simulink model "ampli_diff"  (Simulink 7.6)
settings: Solver=ode15s  StartTime=0.0  StopTime=.2  RelTol=1e-3
StopFcn:
  | close all, clc
  | load  ES_ampli_diff.mat
  | plot(x(1,:),x(2,:))
  | hold on
  | plot(x(1,:),x(3,:))
  | plot(x(1,:),x(4,:))
  | grid
  | title('Tensions d''entrée et de sortie - Ampli différentiel')
  | xlabel('temps')
libraries: fl_lib x13, nesl_utility x4

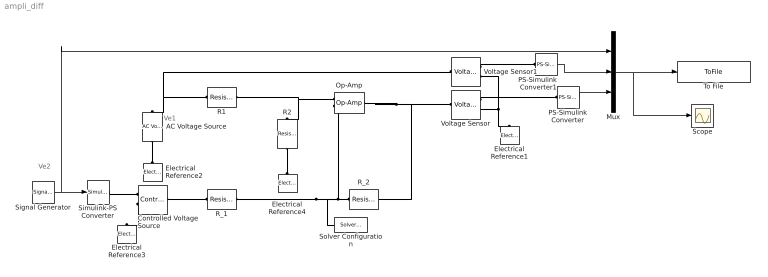
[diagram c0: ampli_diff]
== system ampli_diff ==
  note: Ve1
  note: Ve2
  AC Voltage Source : fl_lib/Electrical/Electrical Sources/AC Voltage Source  DialogController=NetworkEngine.DynNeDlgSource  SystemSampleTime=-1  amp=10 V  shift=2*pi/3 rad  omega=10 Hz  i_Log=off  v_Log=off  LocalVarNames=|current|voltage|power  LocalVarDescs=|Current (A)|Voltage (V)|Power (W)  LocalVarLogging=[0 0 0]
  Controlled Voltage Source : fl_lib/Electrical/Electrical Sources/Controlled Voltage Source  DialogController=NetworkEngine.DynNeDlgSource  SystemSampleTime=-1  i_Log=off  v_Log=off  LocalVarNames=|i|v  LocalVarDescs=|i|v  LocalVarLogging=[0 0]
  Electrical Reference{1..4} (4 alike) : fl_lib/Electrical/Electrical Elements/Electrical Reference  DialogController=NetworkEngine.DynNeDlgSource  SystemSampleTime=-1  i_Log=off  LocalVarNames=|i  LocalVarDescs=|i  LocalVarLogging=[]
  Mux : Mux  Inputs=3
  Op-Amp : fl_lib/Electrical/Electrical Elements/Op-Amp  DialogController=NetworkEngine.DynNeDlgSource  SystemSampleTime=-1  i1_Log=off  v1_Log=off  outI_Log=off  LocalVarNames=|i1|v1|outI  LocalVarDescs=|i1|v1|outI  LocalVarLogging=[0 0 0]
  PS-Simulink Converter : nesl_utility/PS-Simulink Converter  DialogController=NetworkEngine.DynNeUtilDlgSource  SystemSampleTime=-1  PhysicalDomain=network_engine_domain  LeftPortType=input  RightPortType=output  SubClassName=ps_output  Unit=1  AffineConversion=off
  PS-Simulink Converter1 : nesl_utility/PS-Simulink Converter  DialogController=NetworkEngine.DynNeUtilDlgSource  SystemSampleTime=-1  PhysicalDomain=network_engine_domain  LeftPortType=input  RightPortType=output  SubClassName=ps_output  Unit=1  AffineConversion=off
  R1 : fl_lib/Electrical/Electrical Elements/Resistor  DialogController=NetworkEngine.DynNeDlgSource  SystemSampleTime=-1  R=10 kOhm  i_Log=off  v_Log=off  LocalVarNames=|current|voltage|power  LocalVarDescs=|Resistor current (A)|Voltage across resistor (V)|Power (W)  LocalVarLogging=[0 0 0]
  R2 : fl_lib/Electrical/Electrical Elements/Resistor  DialogController=NetworkEngine.DynNeDlgSource  SystemSampleTime=-1  R=10 kOhm  i_Log=off  v_Log=off  LocalVarNames=|current|voltage|power  LocalVarDescs=|Resistor current (A)|Voltage across resistor (V)|Power (W)  LocalVarLogging=[0 0 0]
  R_1 : fl_lib/Electrical/Electrical Elements/Resistor  DialogController=NetworkEngine.DynNeDlgSource  SystemSampleTime=-1  R=10 kOhm  i_Log=off  v_Log=off  LocalVarNames=|current|voltage|power  LocalVarDescs=|Resistor current (A)|Voltage across resistor (V)|Power (W)  LocalVarLogging=[0 0 0]
  R_2 : fl_lib/Electrical/Electrical Elements/Resistor  DialogController=NetworkEngine.DynNeDlgSource  SystemSampleTime=-1  R=10 kOhm  i_Log=off  v_Log=off  LocalVarNames=|current|voltage|power  LocalVarDescs=|Resistor current (A)|Voltage across resistor (V)|Power (W)  LocalVarLogging=[0 0 0]
  Scope : Scope
  Signal Generator : SignalGenerator  Amplitude=8  Frequency=20
  Simulink-PS Converter : nesl_utility/Simulink-PS Converter  DialogController=NetworkEngine.DynNeUtilDlgSource  SystemSampleTime=-1  PhysicalDomain=network_engine_domain  LeftPortType=input  RightPortType=output  SubClassName=ps_input  Unit=1  AffineConversion=off  InputFilterTimeConstant=.001  UdotUserProvided=0
  Solver Configuration : nesl_utility/Solver Configuration  DialogController=NetworkEngine.DynNeUtilDlgSource  SystemSampleTime=-1  PhysicalDomain=network_engine_domain  LeftPortType=input  RightPortType=generic  SubClassName=solver  Accelerate=off  Profile=off  ResidualTolerance=1e-9  MaxNonlinIter=12  MaxModeIter=2  DoFixedCost=off  UseLocalSampling=off  DoDC=off  LinearAlgebra=Sparse  LocalSolverSampleTime=.001  LocalSolverChoice=NE_BACKWARD_EULER_ADVANCER  UseLocalSolver=off
  To File : ToFile  Filename=ES_ampli_diff  MatrixName=x
  Voltage Sensor : fl_lib/Electrical/Electrical Sensors/Voltage Sensor  DialogController=NetworkEngine.DynNeDlgSource  SystemSampleTime=-1  i1_Log=off  v1_Log=off  LocalVarNames=|i1|v1  LocalVarDescs=|i1|v1  LocalVarLogging=[]
  Voltage Sensor1 : fl_lib/Electrical/Electrical Sensors/Voltage Sensor  DialogController=NetworkEngine.DynNeDlgSource  SystemSampleTime=-1  i1_Log=off  v1_Log=off  LocalVarNames=|i1|v1  LocalVarDescs=|i1|v1  LocalVarLogging=[]
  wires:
  Signal Generator/1 -> Simulink-PS Converter/1, Mux/1
  PS-Simulink Converter/1 -> Mux/3
  Mux/1 -> To File/1, Scope/1
  PS-Simulink Converter1/1 -> Mux/2
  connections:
  Op-Amp/LConn1 -- R1/RConn1 -- R2/LConn1
  R_2/LConn1 -- R_1/RConn1 -- Op-Amp/LConn2 -- Solver Configuration/RConn1
  Voltage Sensor1/RConn2 -- Electrical Reference1/LConn1 -- Voltage Sensor/RConn2
  R1/LConn1 -- AC Voltage Source/LConn1 -- Voltage Sensor1/LConn1
  AC Voltage Source/RConn1 -- Electrical Reference2/LConn1
  Controlled Voltage Source/LConn1 -- R_1/LConn1
  Controlled Voltage Source/RConn2 -- Electrical Reference3/LConn1
  Voltage Sensor/RConn1 -- PS-Simulink Converter/LConn1
  Simulink-PS Converter/RConn1 -- Controlled Voltage Source/RConn1
  R2/RConn1 -- Electrical Reference4/LConn1
  Voltage Sensor/LConn1 -- Op-Amp/RConn1 -- R_2/RConn1
  Voltage Sensor1/RConn1 -- PS-Simulink Converter1/LConn1
